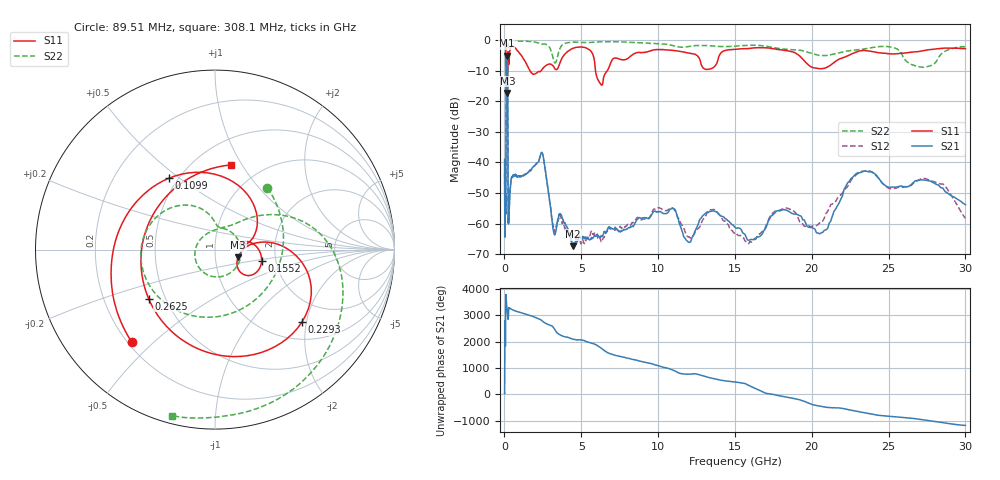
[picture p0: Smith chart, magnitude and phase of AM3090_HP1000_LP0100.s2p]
! Date/Time: Thu, Feb 28, 2019 2:02 PM
! Network Analyzer: Agilent Technologies E8364B Rev: A.07.50.67
! Sweep from 0.010 to 30.000 GHz, 1601 Points, Sweep Type: LOG
! Power Supply: 5.023 V, 0.002 A
# Hz S DB R 50
!freq MagS11 AngS11 MagS21 AngS21 MagS12 AngS12 MagS22 AngS22
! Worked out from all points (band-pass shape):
!   1601 points, 10 MHz to 30 GHz, reference 50 ohm
!   highest |S21| = -5.14 dB at 154.4 MHz (marker M1); lowest = -67.4 dB at 4.48 GHz (marker M2)
!   |S21| within 3 dB of the highest: 121.8 MHz to 199.5 MHz (77.61 MHz wide, 48.3 % of centre)
!   lowest |S11| = -17.3 dB at 189.6 MHz (marker M3), VSWR 1.31, Z = 64.5 - j5.7 ohm
!   |S11| at or under -10 dB: 119.2 MHz to 208.7 MHz (89.46 MHz wide, 54.6 % of centre); 1.648 GHz to 2.393 GHz (745 MHz wide, 36.9 % of centre); 5.925 GHz to 6.697 GHz (771.7 MHz wide, 12.2 % of centre)
!   |S22| runs from -20.2 to -0.2 dB; largest |S21 - S12| = 0.013
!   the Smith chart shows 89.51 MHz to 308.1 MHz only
!   S11 on the Smith chart (normalised r, x): 89.51 MHz: 0.22, -0.43; 109.9 MHz: 0.45, +0.46; 155.2 MHz: 1.68, -0.24; 229.3 MHz: 1.41, -1.89; 262.5 MHz: 0.40, -0.28; 308.1 MHz: 0.73, +0.90
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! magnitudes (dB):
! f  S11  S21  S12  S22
! 10 MHz  -0.3  -39.0  -43.5  -0.4
! 38.04 MHz  -0.5  -59.6  -60.4  -1.3
! 89.51 MHz  -3.2  -48.6  -47.9  -6.9
! 109.9 MHz  -6.5  -18.3  -18.3  -7.6
! 144.7 MHz  -12.9  -5.2  -5.2  -17.3
! 154.4 MHz  -11.5  -5.1  -5.1  -16.4
! 155.2 MHz  -11.4  -5.1  -5.1  -16.4
! 189.6 MHz  -17.3  -6.5  -6.5  -19.9
! 209.6 MHz  -9.6  -12.9  -12.9  -11.8
! 229.3 MHz  -4.0  -40.4  -40.2  -2.8
! 262.5 MHz  -6.8  -60.1  -56.3  -0.8
! 308.1 MHz  -6.4  -55.3  -55.1  -0.4
! 550.5 MHz  -2.0  -44.5  -44.4  -0.2
! 2.084 GHz  -10.8  -40.4  -40.5  -0.8
! 2.482 GHz  -9.5  -37.3  -37.3  -1.3
! 3.22 GHz  -8.9  -63.3  -61.5  -7.0
! 4.48 GHz  -2.7  -67.4  -63.7  -0.7
! 6.234 GHz  -14.2  -64.6  -65.0  -0.6
! 7.926 GHz  -6.3  -61.9  -60.8  -0.7
! 20.41 GHz  -9.3  -63.1  -60.4  -5.0
! 23.48 GHz  -3.4  -42.8  -42.7  -2.9
! 30 GHz  -2.8  -53.8  -58.4  -2.2
